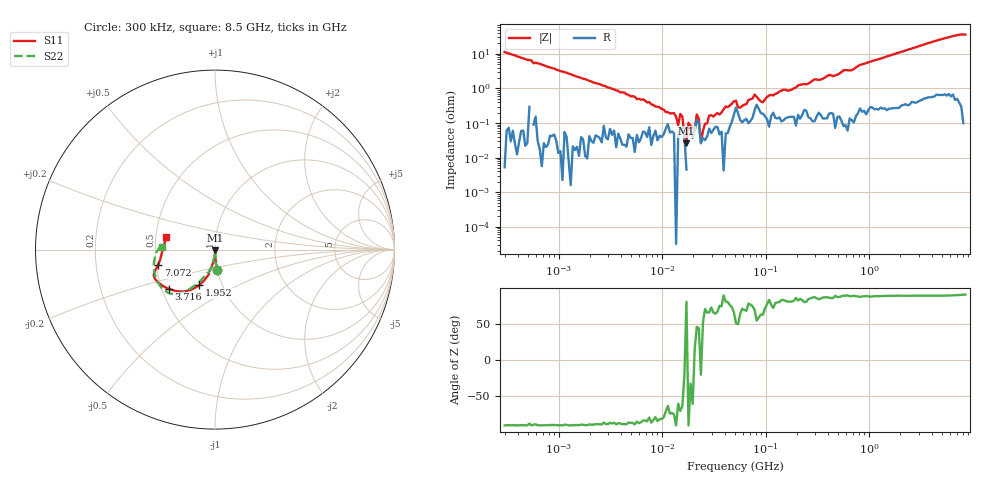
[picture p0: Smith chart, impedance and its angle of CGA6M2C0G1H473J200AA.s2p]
! S-parameter Generated by TDK Corporation
! Copyright(C) 2015 TDK Corporation.
! All Rights Reserved.
! TDK P/N: CGA6M2C0G1H473J200AA (Multilayer Ceramic Chip Capacitors)
! Property: C=47nF
! Size(LxWxT): 3.2x2.5x2mm, 0.126x0.098x0.079inches
! Model Type: s2p (Touchstone File Format Version 1.0)
! Frequency: DC=Yes Start=0.3MHz Stop=8500MHz 225points Log-sweep
! Note:
! Model Generated on Jun. 23, 2015
! Hash(MD5):
! Port Assignments:
!  1 ---| |--- 2
! Applicable Conditions:
!  Temperature = 25 degC
!  DC Bias Voltage = 0 V
!  Small Signal Operation
! Terms and conditions regarding TDK Simulation Models
! (1)This simulation model is being provided solely for informational purposes. Please refer to the specifications of the products in terms of detailed characteristics of such products.
! (2)In no event shall TDK Corporation of any of its subsidiaries be liable for any loss or damage arising, directly or indirectly,
!  From any information contained in this simulation model, including, but not limited to loss or damages arising from any inaccuracies, omissions or errors in connection with such information.
! (3)Any and all copyrights on this simulation model are owned by TDK Corporation.
!  Duplication or redistribution of this simulation model without prior written permission from TDK Corporation is prohibited.
! (4)This simulation model is subject to any modification or change without any prior notice.
! (5)Neither TDK Corporation nor any of its subsidiaries shall make any warranty, express or implied,
!  Including but not limited to the correctness, implied warranties of merchantability and fitness for a particular purpose with respect to this simulation models.
! (6)The use of this simulation model shall be deemed to have consented to the terms and conditions hereof.
# MHz S MA R 50
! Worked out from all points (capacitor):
!   224 points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, 300 kHz to 8.5 GHz, reference 50 ohm
!   read as one part in series: C = 47.1 nF near 314.1 kHz
!   lowest |Z| = 26.2 mohm at 17.14 MHz (marker M1)
!   series resonance near 16.68 MHz, so ESL is about 1.9 nH
!   S11 on the Smith chart (normalised r, x): 300 kHz: 1.00, -0.23; 1.952 GHz: 0.78, -0.32; 3.716 GHz: 0.54, -0.27; 7.072 GHz: 0.51, -0.10; 8.5 GHz: 0.57, +0.09
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0.3  0.1121 -83.7  0.9937 6.5  0.9933 6.5  0.112 -83.4
1.72111  0.01957 -86.6  0.9996 1.0  0.9993 1.1  0.01968 -89.5
9.430415  0.004561 -83.9  0.9999 0.1  0.999 0.1  0.004363 -88.1
17.1428  0.00358 -86.8  1 -0.3  0.9999 -0.2  0.003576 -93.1
20.60362  0.003532 -78.0  0.9996 -0.2  0.9989 -0.2  0.003861 -86.1
21.57293  0.003873 -81.6  0.9983 -0.4  0.9978 -0.3  0.00331 -82.9
23.65048  0.0036 -85.3  0.9998 -0.2  0.9996 -0.2  0.003969 -88.5
31.16253  0.003692 -83.4  0.9991 -0.4  0.9991 -0.3  0.004249 -86.1
47.13265  0.004657 -80.0  0.9991 -0.7  0.9981 -0.6  0.004445 -80.5
51.67171  0.006269 -62.2  0.9972 -0.7  0.9971 -0.7  0.005999 -65.5
54.10262  0.007113 -74.6  0.9982 -0.6  0.998 -0.6  0.007138 -76.8
71.28712  0.007153 -85.5  0.9979 -1.0  0.9991 -0.9  0.007265 -82.8
78.15234  0.008232 -78.0  0.9972 -1.2  0.9972 -1.1  0.007544 -75.4
89.70948  0.01144 -81.6  0.9994 -1.1  0.9957 -1.0  0.01087 -85.1
283.1228  0.03067 -92.3  0.9979 -3.7  0.9973 -3.6  0.03018 -93.6
678.1388  0.07523 -97.9  0.9944 -8.2  0.9927 -8.1  0.0742 -100.2
1551.304  0.174 -108.3  0.9777 -20.4  0.9779 -20.3  0.1746 -113.1
1952.199  0.2153 -113.8  0.9688 -25.7  0.9684 -25.5  0.2171 -118.0
3715.7  0.3374 -139.6  0.9276 -46.7  0.9252 -46.6  0.3397 -133.3
5126.239  0.3722 -154.1  0.9129 -61.9  0.9093 -61.7  0.3668 -147.3
7072.242  0.328 -165.0  0.9186 -82.8  0.9182 -82.7  0.3272 -177.1
8500  0.2797 165.5  0.9243 -100.7  0.9294 -100.3  0.2957 176.7
